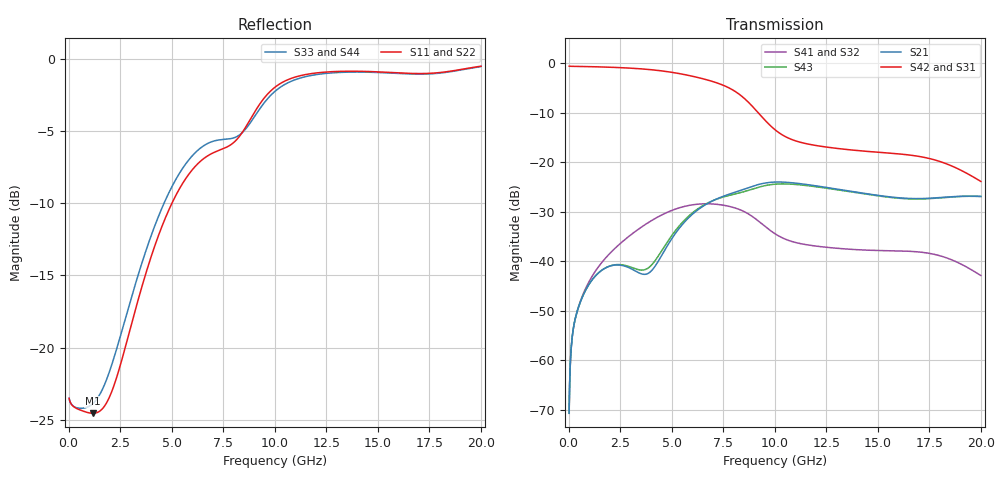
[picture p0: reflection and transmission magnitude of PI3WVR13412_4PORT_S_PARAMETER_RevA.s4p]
! NPort=4 DATA=800 NOISE=0 GROUPDELAY=0 COMPLEX_DATAFORMAT=POLAR
! NumOfBlock=1 NumOfParam=0
! .MODEL Smodel S TSTONEFILE=PI3WVR13412_4PORT_S_PARAMETER_RevA.s4p TYPE=S
!  -- The above .MODEL line can be used for the S element in the netlist.
! PORT DEFINITION
! PORT1 = INPUT+
! PORT2 = INPUT-
! PORT3 = OUTPUT+
! PORT4 = OUTPUT-
# Hz S MA R  50
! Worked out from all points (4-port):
!   800 points, 25 MHz to 20 GHz, reference 50 ohm
!   strongest paths, dB at 25 MHz, 5.025 GHz, 10.03 GHz, 15.03 GHz, 20 GHz:
!     S42: -0.6, -1.9, -13.5, -18.0, -23.9
!     S31: -0.6, -1.9, -13.5, -18.0, -23.9
!     S21: -70.6, -35.3, -24.0, -26.7, -26.9
!     S43: -70.6, -34.7, -24.4, -26.8, -26.9
!     S41: -70.7, -29.7, -34.5, -37.8, -42.9
!     S32: -70.7, -29.7, -34.5, -37.8, -42.9
!   lowest |S11| = -24.6 dB at 1.175 GHz (marker M1), VSWR 1.13, Z = 56.2 - j0.845 ohm
!   |S11| at or under -10 dB: start of sweep to 5.013 GHz
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2.5e7  0.06671 -2.1  0.0002936 86.1  0.9298 -0.7  0.0002922 86.0
       0.0002936 86.1  0.06671 -2.1  0.0002922 86.0  0.9298 -0.7
       0.9298 -0.7  0.0002922 86.0  0.06671 -1.9  0.0002936 86.1
       0.0002922 86.0  0.9298 -0.7  0.0002936 86.1  0.06671 -1.9
3e8  0.06201 -4.9  0.002508 65.0  0.925 -6.5  0.00251 64.5
     0.002508 65.0  0.06201 -4.9  0.00251 64.5  0.925 -6.5
     0.9251 -6.5  0.002511 64.5  0.06219 -2.3  0.002507 65.2
     0.002511 64.5  0.9251 -6.5  0.002507 65.2  0.06219 -2.3
1.175e9  0.05917 -7.3  0.006631 58.1  0.9182 -24.9  0.007246 55.7
         0.006631 58.1  0.05917 -7.3  0.007246 55.7  0.9182 -24.9
         0.9183 -24.9  0.007246 55.7  0.06393 2.1  0.00663 58.8
         0.007246 55.7  0.9183 -24.9  0.00663 58.8  0.06393 2.1
4e9  0.206 -1.7  0.007942 77.5  0.8564 -86.7  0.02555 0.8
     0.007942 77.5  0.206 -1.7  0.02555 0.8  0.8564 -86.7
     0.8566 -86.7  0.02556 0.8  0.2436 -2.7  0.009049 77.9
     0.02556 0.8  0.8566 -86.7  0.009049 77.9  0.2436 -2.7
6.85e9  0.4662 -48.8  0.03939 72.4  0.664 -155.8  0.03795 -82.4
        0.03939 72.4  0.4662 -48.8  0.03795 -82.4  0.664 -155.8
        0.6643 -155.7  0.03796 -82.3  0.5134 -53.2  0.03964 67.5
        0.03796 -82.3  0.6643 -155.7  0.03964 67.5  0.5134 -53.2
8.875e9  0.6278 -59.2  0.05664 44.1  0.373 148.6  0.02864 -143.5
         0.05664 44.1  0.6278 -59.2  0.02864 -143.5  0.373 148.6
         0.3732 148.7  0.02865 -143.4  0.6093 -64.2  0.05309 41.6
         0.02865 -143.4  0.3732 148.7  0.05309 41.6  0.6093 -64.2
2e10  0.9436 -127.3  0.04513 -30.1  0.06379 21.6  0.007164 45.0
      0.04513 -30.1  0.9436 -127.3  0.007164 45.0  0.06379 21.6
      0.06387 21.8  0.007173 45.2  0.9407 -127.3  0.04502 -29.7
      0.007173 45.2  0.06387 21.8  0.04502 -29.7  0.9407 -127.3
